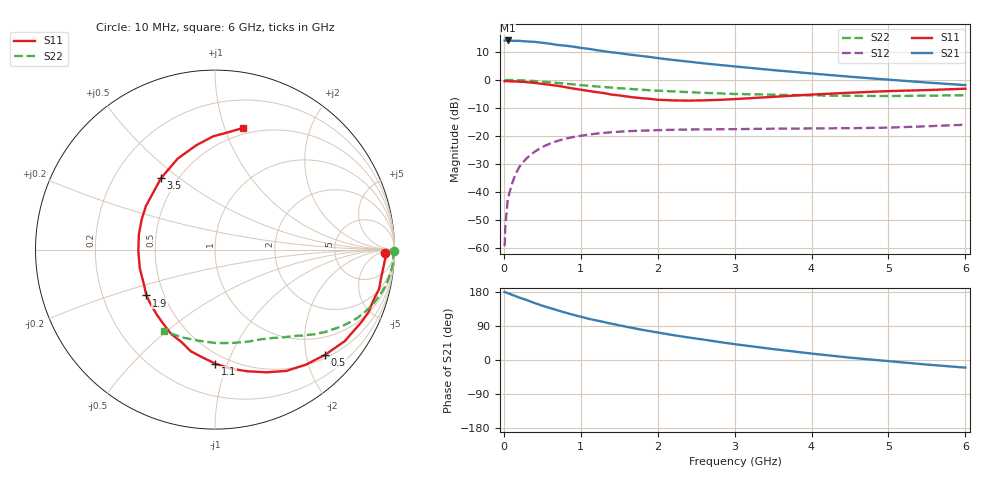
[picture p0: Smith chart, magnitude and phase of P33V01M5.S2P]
! SIEMENS Small Signal Semiconductors
! BFP181
! Si NPN RF Bipolar Junction Transistor in SOT143
! VCE = 3 V  IC = 1.5 mA
! Common Emitter S-Parameters:  March  1996
# GHz  S  MA  R  50
!  f  S11  S21  S12  S22
! GHz  MAG  ANG  MAG  ANG  MAG  ANG  MAG  ANG
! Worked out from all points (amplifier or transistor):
!   36 points, 10 MHz to 6 GHz, reference 50 ohm
!   highest |S21| = 14.0 dB at 50 MHz (marker M1)
!   |S21| within 3 dB of that: start of sweep to 1.109 GHz
!   unconditionally stable (mu >= 1): 2.713 GHz to end of sweep
!   at 250 MHz: K = 0.11, MSG = 21.5 dB, |S12| = -29.3 dB
!   at 1.4 GHz: K = 0.58, MSG = 14.2 dB, |S12| = -18.6 dB
!   at 6 GHz: K = 1.18, MAG = 4.5 dB, |S12| = -16.0 dB
!   S11 on the Smith chart (normalised r, x): 10 MHz: 33, -10; 500 MHz: 0.57, -2.38; 1.1 GHz: 0.43, -0.91; 1.9 GHz: 0.40, -0.26; 3.5 GHz: 0.41, +0.43; 6 GHz: 0.44, +1.16
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0.01  0.9465 -1.0  5.009 179.5  0.0011 84.2  0.998 -0.4
0.02  0.954 -2.0  5.007 179.0  0.0025 92.3  0.9909 -0.8
0.05  0.9472 -4.1  5.028 176.3  0.0074 89.6  0.9946 -2.0
0.1  0.9393 -9.0  4.967 172.6  0.0135 81.8  0.9947 -4.1
0.2  0.9264 -18.0  4.963 164.9  0.028 79.5  0.9846 -8.1
0.4  0.8847 -35.2  4.751 150.3  0.0527 68.4  0.9523 -15.7
0.5  0.8484 -43.7  4.578 143.3  0.0639 62.8  0.9296 -19.3
0.6  0.8173 -51.6  4.4 137.2  0.0736 58.2  0.9054 -22.5
0.8  0.7421 -67.1  4.061 125.0  0.0898 50.1  0.8572 -28.0
0.9  0.7021 -75.0  3.902 119.4  0.0963 46.3  0.8319 -30.5
1.1  0.6358 -89.8  3.576 108.9  0.1064 40.0  0.7854 -34.8
1.3  0.5826 -103.3  3.234 100.2  0.114 34.4  0.746 -38.6
1.5  0.5292 -117.7  2.993 91.5  0.1197 30.0  0.7104 -41.8
1.7  0.486 -132.0  2.753 83.5  0.1236 26.4  0.6805 -44.8
1.9  0.4599 -146.3  2.551 76.1  0.126 23.1  0.6537 -47.5
2.2  0.4316 -166.3  2.262 65.7  0.1295 19.3  0.6237 -51.5
2.8  0.4412 158.1  1.845 47.5  0.1322 14.0  0.5752 -59.8
3.5  0.4987 127.1  1.493 28.8  0.1355 10.2  0.5448 -70.4
4  0.5479 112.3  1.3 17.0  0.1367 8.5  0.5292 -79.6
4.5  0.5909 100.1  1.139 6.2  0.1383 7.4  0.5205 -89.7
5.5  0.6585 83.4  0.897 -12.1  0.1495 7.8  0.5232 -111.0
6  0.6963 76.9  0.807 -20.1  0.1593 6.8  0.5341 -122.0
